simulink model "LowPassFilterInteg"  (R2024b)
settings: Solver=FixedStepAuto  StartTime=0.0  StopTime=0.3  FixedStep=1e-3  RelTol=1e-3

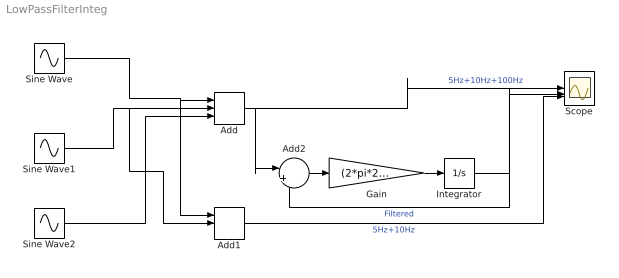
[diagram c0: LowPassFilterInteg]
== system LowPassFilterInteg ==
  Add : Sum  Inputs=+++
  Add1 : Sum  Inputs=+++
  Add2 : Sum  Inputs=|+-
  Gain : Gain  Gain=(2*pi*20)
  Integrator : Integrator
  Scope : Scope  NumInputPorts=3
  Sine Wave : Sin  Frequency=2 * pi * 5  SampleTime=0
  Sine Wave1 : Sin  Frequency=2 * pi * 10  Phase=pi/4  SampleTime=0
  Sine Wave2 : Sin  Frequency=2 * pi * 100  Phase=pi/2  SampleTime=0
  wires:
  Sine Wave/1 -> Add1/1, Add/1
  Sine Wave1/1 -> Add1/2, Add/2
  Sine Wave2/1 -> Add/3
  Add/1 -> Scope/1, Add2/1  "5Hz+10Hz+100Hz"
  Integrator/1 -> Add2/2, Scope/2  "Filtered"
  Add1/1 -> Scope/3  "5Hz+10Hz"
  Add2/1 -> Gain/1
  Gain/1 -> Integrator/1
